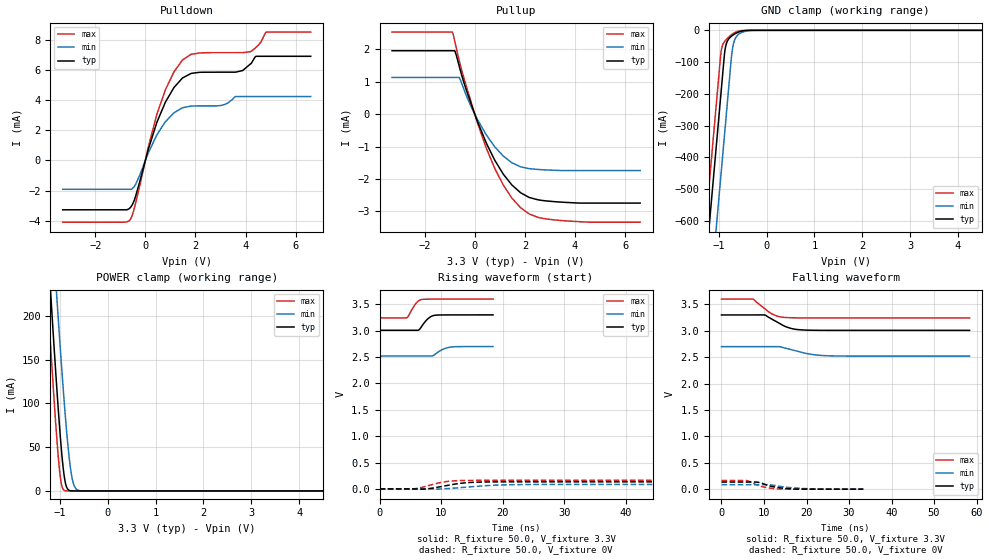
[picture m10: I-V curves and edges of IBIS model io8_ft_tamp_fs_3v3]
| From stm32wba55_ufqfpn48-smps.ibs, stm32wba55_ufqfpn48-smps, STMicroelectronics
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[Model]   io8_ft_tamp_fs_3v3
Model_type I/O
Polarity   Non-Inverting
Enable   Active-Low
| CAP_THRESHOLD on pad IOFT is "UDTCAPC" :
| Rising=30.0% of vddiom   Falling=70.0% of vddiom
| C_comp min and max val. don't necessarily correlate with the min and max pvt
| but are the smallest and greatest pad capacitance found.
| var   typ   min   max
C_comp   8.02920pF  7.67210pF  8.31249pF
|C_comp_pullup   5.44714pF  5.17604pF  5.56514pF
|C_comp_pulldown   2.58206pF  2.49607pF  2.74735pF
Vinl = 1.35V
Vinh = 1.8V
Vmeas = 1.65V   | Reference voltage for timing measurements
Cref  = 50.0pF   | Timing specification test load capacitance value
Rref  = 1.0MOhm   | Timing specification test load resistance value
Vref  = 1.815V   | Timing specification test load voltage
[Model Spec]
| TIME_THRESHOLD on pin ZIV33SW is "CMOS" :
| Rising=50.0% of VDDV33SW   Falling=50.0% of VDDV33SW
Vinl 1.28450V 1.07650V 1.38450V
Vinh 1.79550V 1.49050V 1.94250V
| variable   typ   min   max
[Temperature Range] 25.0 140.0 -40.0
| variable   typ   min   max
[Voltage Range] 3.3V 2.7V 3.6V
| variable   typ   min   max
[POWER Clamp Reference] 3.3V 2.7V 3.6V
| variable   typ   min   max
[GND Clamp Reference] 0V 0V 0V
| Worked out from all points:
|   slope of the pulldown table from 0 to 0.495 V, typ, clamps not added: 186 ohm
|   slope of the pullup table from 0 to 0.495 V, typ, clamps not added: 523 ohm
|   GND clamp passes 1 mA (typ) near -0.47 V on its own axis
|   POWER clamp passes 1 mA (typ) near -0.81 V on its own axis
|   rising waveform, R_fixture 50.0, V_fixture 3.3V: 20-80 % time 1.27ns typ, 1.6ns min, 1.13ns max; typ from 3.01 V to 3.3 V
|   falling waveform, R_fixture 50.0, V_fixture 3.3V: 20-80 % time 4.1ns typ, 5.6ns min, 3.53ns max; typ from 3.3 V to 3.01 V
|   rising waveform, R_fixture 50.0, V_fixture 0V: 20-80 % time 4.09ns typ, 5.95ns min, 3.46ns max; typ from 0 V to 0.135 V
|   falling waveform, R_fixture 50.0, V_fixture 0V: 20-80 % time 4ns typ, 5.62ns min, 3.42ns max; typ from 0.135 V to 0 V
[POWER Clamp]
-3.3V     2.246A     2.279A     2.182A
-1.26V    287mA      389.3mA    225.1mA
-1.19V    224.6mA    328.4mA    163.1mA
-1.06V    114.5mA    218.6mA    57.35mA
-1.02V    83.5mA     186.1mA    30.99mA
-980mV    55.21mA    154.6mA    11.87mA
-900mV    13.79mA    95.47mA    485.6uA
-820mV    1.189mA    45.7mA     11.82uA
-760mV    138.8uA    19.43mA    717.3nA
-690mV    10.88uA    4.64mA     27.56nA
-600mV    410.2nA    489.5uA    725pA
6.6V      0A         0A         0A
[GND Clamp]
-3.3V     -4.191A    -4.447A    -4.059A
-1.59V    -1.284A    -1.54A     -1.152A
-1.25V    -705.7mA   -962.2mA   -574mA
-960mV    -212.7mA   -469.2mA   -81mA
-950mV    -195.7mA   -452.2mA   -68.07mA
-880mV    -77.2mA    -333.2mA   -36.04mA
-850mV    -48.09mA   -282.2mA   -30.39mA
-720mV    -17.06mA   -67.51mA   -12.51mA
-680mV    -12.85mA   -36.48mA   -8.6mA
-630mV    -8.529mA   -19.6mA    -4.86mA
-220mV    -490.4nA   -42.83uA   -18.74nA
6.6V      5.835nA    6.044uA    3.958nA
| variable   typ   min   max
[Pullup Reference] 3.3V 2.7V 3.6V
| variable   typ   min   max
[Pulldown Reference] 0V 0V 0V
[Pullup]
-3.3V     1.956mA    1.132mA    2.53mA
-890mV    1.956mA    1.132mA    2.523mA
-790mV    1.939mA    1.132mA    2.221mA
-610mV    1.448mA    1.114mA    1.613mA
-90mV     195.3uA    143.2uA    228.7uA
460mV     -891.2uA   -639.5uA   -1.049mA
800mV     -1.423mA   -1.009mA   -1.677mA
1.14V     -1.853mA   -1.295mA   -2.188mA
1.83V     -2.424mA   -1.624mA   -2.886mA
2.51V     -2.639mA   -1.705mA   -3.178mA
3.17V     -2.697mA   -1.73mA    -3.259mA
6.6V      -2.742mA   -1.738mA   -3.331mA
[Pulldown]
-3.3V     -3.274mA   -1.917mA   -4.095mA
-610mV    -3.144mA   -1.917mA   -3.932mA
-390mV    -2.378mA   -1.591mA   -2.836mA
460mV     2.524mA    1.696mA    3.053mA
800mV     3.862mA    2.563mA    4.678mA
1.48V     5.456mA    3.486mA    6.647mA
3.01V     5.842mA    3.632mA    7.136mA
3.6V      5.844mA    4.228mA    7.136mA
4.19V     6.383mA    4.228mA    7.196mA
4.41V     6.889mA    4.228mA    7.475mA
4.83V     6.894mA    4.228mA    8.498mA
6.6V      6.894mA    4.228mA    8.498mA
[Ramp]
dV/dt_r 80.90749mV/4.07268ns 51.28754mV/5.94334ns 98.35263mV/3.38777ns
dV/dt_f 175.29312mV/4.09732ns 108.33331mV/5.58653ns 214.11123mV/3.52657ns
R_load = 50.0
| Removed startup time: 0s 0s 0s  .
| Removed end time: 18.4ns.
[Rising Waveform]
R_fixture   = 50.0
V_fixture   = 3.3V
V_fixture_min = 2.7V
V_fixture_max = 3.6V
0s        3.008V     2.519V     3.243V
4.4ns     3.008V     2.519V     3.245V
5.85ns    3.008V     2.519V     3.512V
6.35ns    3.015V     2.519V     3.569V
6.8ns     3.079V     2.519V     3.591V
7.85ns    3.228V     2.519V     3.598V
8.85ns    3.29V      2.542V     3.599V
10.15ns   3.298V     2.641V     3.6V
11.55ns   3.3V       2.69V      3.6V
18.4ns    3.3V       2.7V       3.6V
| Removed startup time: 0s 0s 0s  .
| Removed end time: 58.35ns.
[Falling Waveform]
R_fixture   = 50.0
V_fixture   = 3.3V
V_fixture_min = 2.7V
V_fixture_max = 3.6V
0s        3.3V       2.7V       3.6V
7.45ns    3.3V       2.7V       3.599V
10.3ns    3.298V     2.7V       3.412V
12.1ns    3.21V      2.701V     3.311V
13.5ns    3.147V     2.7V       3.269V
15.05ns   3.081V     2.671V     3.253V
18ns      3.022V     2.61V      3.245V
21.45ns   3.01V      2.55V      3.243V
25.05ns   3.008V     2.527V     3.243V
58.35ns   3.008V     2.519V     3.243V
| Removed startup time: 0s 0s 0s  .
| Removed end time: 58.35ns.
[Rising Waveform]
R_fixture   = 50.0
V_fixture   = 0V
V_fixture_min = 0V
V_fixture_max = 0V
0s        162.8nV    4.5uV      290.6nV
5ns       592.9nV    4.496uV    -4.389mV
5.95ns    36.68uV    4.553uV    7.752mV
7.55ns    325.1uV    9.527uV    51.62mV
9.65ns    37.78mV    -2.109mV   115.7mV
10.75ns   61.07mV    4.605mV    138.6mV
13.4ns    110.2mV    27.48mV    159.6mV
16.95ns   131.6mV    59.51mV    163.6mV
22.15ns   134.7mV    81.55mV    163.9mV
58.35ns   134.8mV    85.48mV    163.9mV
| Removed startup time: 0s 0s 0s  .
| Removed end time: 33.35ns.
[Falling Waveform]
R_fixture   = 50.0
V_fixture   = 0V
V_fixture_min = 0V
V_fixture_max = 0V
0s        134.9mV    85.5mV     163.9mV
5.9ns     134.9mV    85.5mV     162.7mV
6.9ns     134.9mV    85.5mV     137mV
8.35ns    134.3mV    85.5mV     77.77mV
9.4ns     114.4mV    85.5mV     51.36mV
11ns      67.97mV    85.48mV    25.24mV
13.5ns    28.5mV     56.61mV    3.307mV
17.05ns   3.292mV    23.87mV    179.7uV
21.15ns   146.6uV    6.27mV     23.82uV
33.35ns   996.2nV    26.32uV    845.4nV
